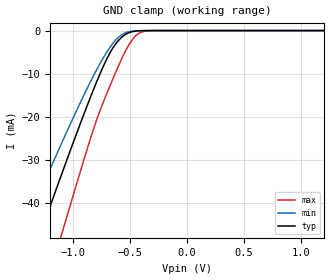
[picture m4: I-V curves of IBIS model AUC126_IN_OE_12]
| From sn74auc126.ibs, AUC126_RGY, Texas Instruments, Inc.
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[Model]   AUC126_IN_OE_12
Model_type  Input
Vinl=0.385
Vinh=0.845
| variable   typ   min   max
C_comp   2.65pF   2.25pF   3.08pF
[Temperature Range]   40   100   -40
| Ambient temperature   25   85   -40
[Voltage range]   1.2   1.1   1.3
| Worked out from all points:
|   GND clamp passes 1 mA (typ) near -0.55 V on its own axis
[GND Clamp]
| AUC126_IN_OE_12
|   Voltage   I(typ)   I(min)   I(max)
-3.6V     -222.6mA   -186.3mA   -267.8mA
-1.45V    -59.34mA   -47.37mA   -78.58mA
-1.405V   -55.97mA   -44.58mA   -74.57mA
-1.275V   -46.26mA   -36.62mA   -62.96mA
-1.11V    -34.1mA    -26.74mA   -48.2mA
-1.075V   -31.55mA   -24.68mA   -45.07mA
-835mV    -14.65mA   -11.24mA   -24.05mA
-695mV    -6.117mA   -4.635mA   -14.06mA
-575mV    -1.603mA   -1.004mA   -6.664mA
-440mV    -95.43uA   -45.4uA    -977.4uA
-320mV    -2.85uA    -1.752uA   -25.53uA
1.2V      140.4pA    230.5pA    130.8pA
